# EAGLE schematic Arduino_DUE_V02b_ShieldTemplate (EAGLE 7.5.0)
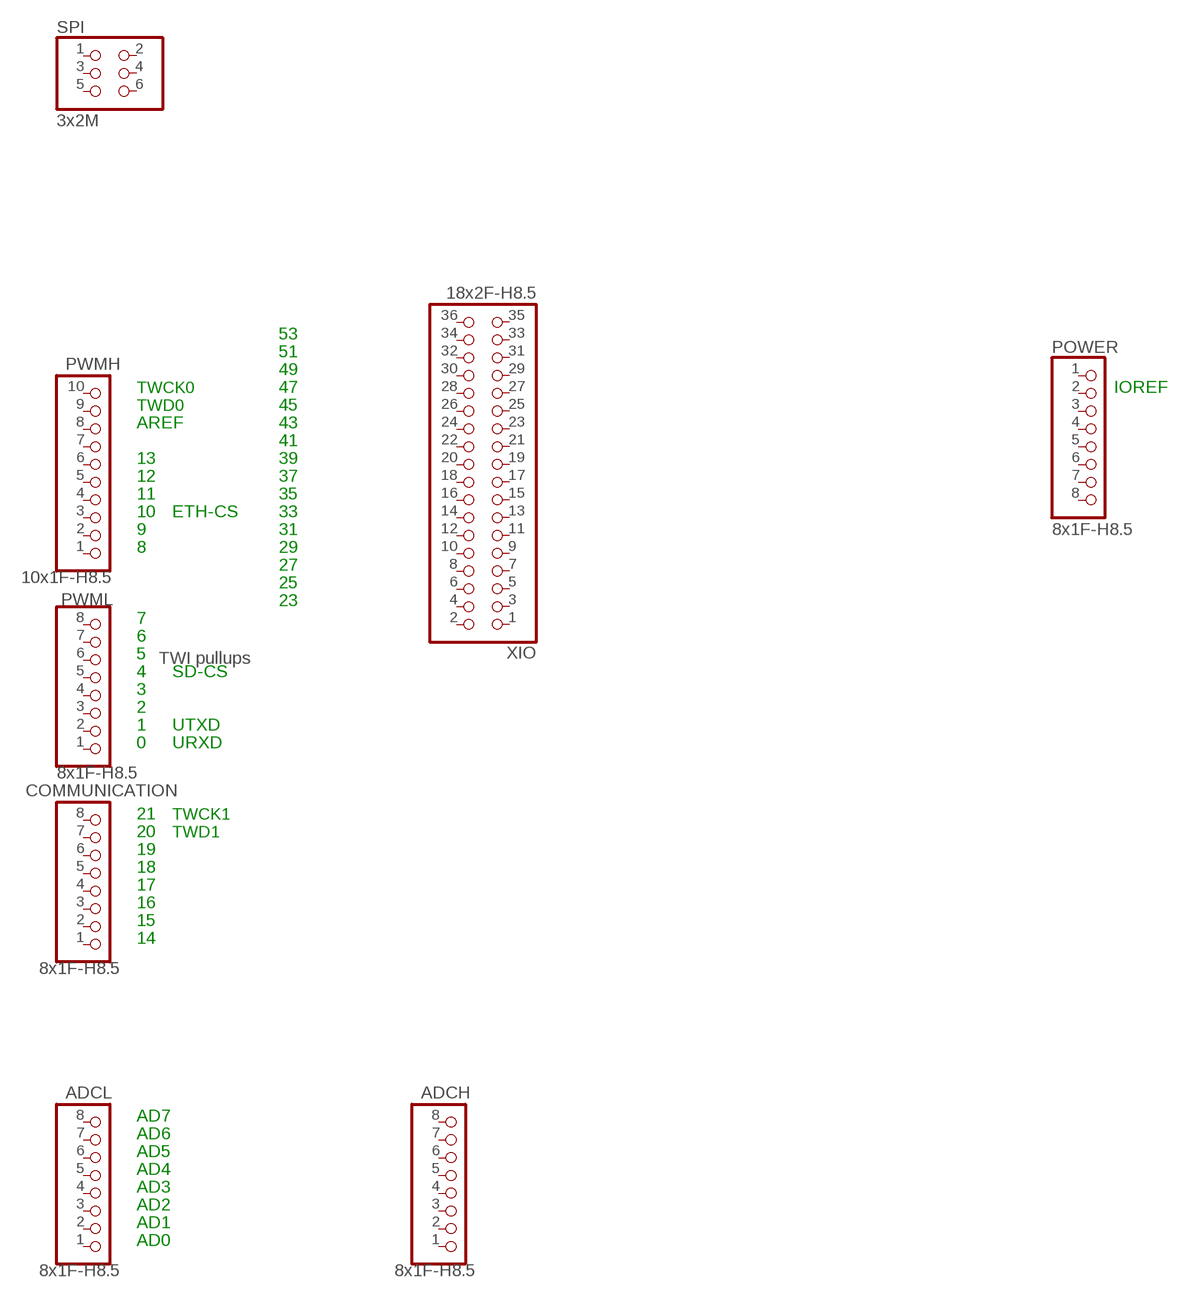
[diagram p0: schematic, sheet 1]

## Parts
ADCH  8x1F-H8.5  PINHD-1X8  [1X08]
ADCL  8x1F-H8.5  PINHD-1X8  [1X08]
COMMUNICATION  8x1F-H8.5  PINHD-1X8  [1X08]
POWER  8x1F-H8.5  PINHD-1X8  [1X08]
PWMH  10x1F-H8.5  PINHD-1X10  [1X10]
PWML  8x1F-H8.5  PINHD-1X8  [1X08]
SPI  3x2M  PINHD-2X3  [2X03]
XIO  18x2F-H8.5  PINHD-2X18  [2X18]
Unconnected: ADCH.1 ADCH.2 ADCH.3 ADCH.4 ADCH.5 ADCH.6 ADCH.7 ADCH.8 ADCL.1 ADCL.2 ADCL.3 ADCL.4 ADCL.5 ADCL.6 ADCL.7 ADCL.8 COMMUNICATION.1 COMMUNICATION.2 COMMUNICATION.3 COMMUNICATION.4 COMMUNICATION.5 COMMUNICATION.6 COMMUNICATION.7 COMMUNICATION.8 POWER.1 POWER.2 POWER.3 POWER.4 POWER.5 POWER.6 POWER.7 POWER.8 PWMH.1 PWMH.2 PWMH.3 PWMH.4 PWMH.5 PWMH.6 PWMH.7 PWMH.8 PWMH.9 PWMH.10 PWML.1 PWML.2 PWML.3 PWML.4 PWML.5 PWML.6 PWML.7 PWML.8 SPI.1 SPI.2 SPI.3 SPI.4 SPI.5 SPI.6 XIO.1 XIO.2 XIO.3 XIO.4 XIO.5 XIO.6 XIO.7 XIO.8 XIO.9 XIO.10 XIO.11 XIO.12 XIO.13 XIO.14 XIO.15 XIO.16 XIO.17 XIO.18 XIO.19 XIO.20 XIO.21 XIO.22 XIO.23 XIO.24 XIO.25 XIO.26 XIO.27 XIO.28 XIO.29 XIO.30 XIO.31 XIO.32 XIO.33 XIO.34 XIO.35 XIO.36

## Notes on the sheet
- 53
- 51
- 49
- TWCK0 | 47 | IOREF
- TWD0 | 45
- AREF | 43
- 41
- 13 | 39
- 12 | 37
- 11 | 35
- 10 | ETH-CS | 33
- 9 | 31
- 8 | 29
- 27
- 25
- 23
- 7
- 6
- 5 | TWI pullups
- 4 | SD-CS
- 3
- 2
- 1 | UTXD
- 0 | URXD
- 21 | TWCK1
- 20 | TWD1
- 19
- 18
- 17
- 16
- 15
- 14
- AD7
- AD6
- AD5
- AD4
- AD3
- AD2
- AD1
- AD0

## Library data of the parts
ADCH ADCL COMMUNICATION POWER PWML = SmartPrj:PINHD-1X8: PIN HEADER
PWMH = SmartPrj:PINHD-1X10: PIN HEADER
SPI = SmartPrj:PINHD-2X3: PIN HEADER
XIO = SmartPrj:PINHD-2X18: PIN HEADER

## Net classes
0 default: width 0.203 mm, drill 0.305 mm, clearance 0.203 mm
1 USB: drill 0.406 mm, clearance 0.203 mm to class 0, clearance 0.406 mm
2 gnd: width 0.305 mm, drill 0.406 mm, clearance 0.203 mm to class 0, clearance 0.203 mm
3 usbvcc: width 0.61 mm, drill 0.508 mm, clearance 0.203 mm to class 0, clearance 0.254 mm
